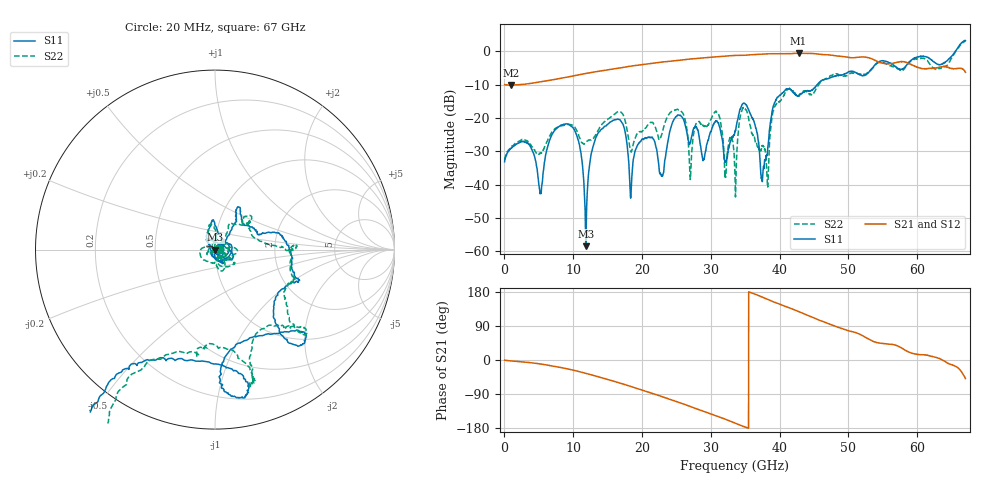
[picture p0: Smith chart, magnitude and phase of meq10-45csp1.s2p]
!Keysight Technologies,N5247B,US58420632,A.14.00.23
!Date: Monday, March 14, 2022 13:46:42
!Correction: S22(C  2-Port  )
!S42(C  2-Port  )
!S24(C  2-Port  )
!S44(C  2-Port  )
!S2P File: Measurement: :
# Hz S  dB  R 50
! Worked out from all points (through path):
!   3350 points, 20 MHz to 67 GHz, reference 50 ohm
!   highest |S21| = -0.62 dB at 42.76 GHz (marker M1); lowest = -10.2 dB at 920 MHz (marker M2)
!   group delay of S21, straight-line fit = 17.3 ps
!   lowest |S11| = -58.5 dB at 11.82 GHz (marker M3), VSWR 1.00, Z = 50.1 - j0.031 ohm
!   |S11| at or under -10 dB: start of sweep to 45.47 GHz
!   |S22| runs from -43.7 to 3.1 dB; largest |S21 - S12| = 0.0054
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2e7  -33.14 3.7  -10.05 -0.2  -10.06 -0.3  -32.61 2.0
9.2e8  -29.13 16.9  -10.16 -2.4  -10.15 -2.5  -28.73 15.4
5.22e9  -42.53 -2.5  -9.20 -10.4  -9.20 -10.4  -30.58 -0.5
7.92e9  -22.61 -17.5  -8.24 -18.9  -8.24 -18.9  -22.56 -2.7
1.12e10  -31.91 60.3  -6.93 -32.2  -6.93 -32.2  -27.39 11.0
1.182e10  -58.47 -15.0  -6.69 -35.2  -6.69 -35.2  -27.32 -17.0
1.306e10  -27.30 -89.7  -6.24 -41.4  -6.24 -41.4  -25.66 -48.5
1.556e10  -21.06 -18.7  -5.43 -54.3  -5.43 -54.4  -19.60 -18.1
1.836e10  -43.76 149.6  -4.49 -69.8  -4.49 -69.9  -29.90 -31.5
2.236e10  -32.86 -24.4  -3.40 -93.2  -3.40 -93.3  -25.80 -43.4
2.55e10  -19.28 -22.7  -2.71 -112.9  -2.72 -112.9  -17.91 -34.2
2.704e10  -27.26 91.6  -2.35 -123.0  -2.36 -123.0  -37.95 87.0
3.082e10  -21.07 -59.9  -1.71 -147.7  -1.71 -147.8  -18.16 -68.0
3.352e10  -23.95 54.2  -1.28 -166.6  -1.29 -166.6  -38.66 -152.5
3.476e10  -15.58 93.7  -1.24 -175.4  -1.24 -175.6  -16.95 99.5
3.75e10  -38.50 -109.3  -0.89 165.7  -0.90 165.6  -28.54 -166.9
3.826e10  -29.24 7.5  -0.81 159.8  -0.81 159.7  -40.43 -51.3
3.936e10  -15.14 52.4  -0.78 151.8  -0.78 151.7  -16.35 60.8
4.276e10  -13.47 41.2  -0.62 127.9  -0.63 127.6  -13.38 42.2
4.468e10  -11.68 18.6  -0.70 113.6  -0.69 113.3  -13.05 26.6
5.584e10  -3.34 -42.9  -3.79 42.1  -3.79 41.9  -4.16 -44.0
6.7e10  3.16 -116.5  -6.33 -48.9  -6.33 -49.0  3.06 -115.6
